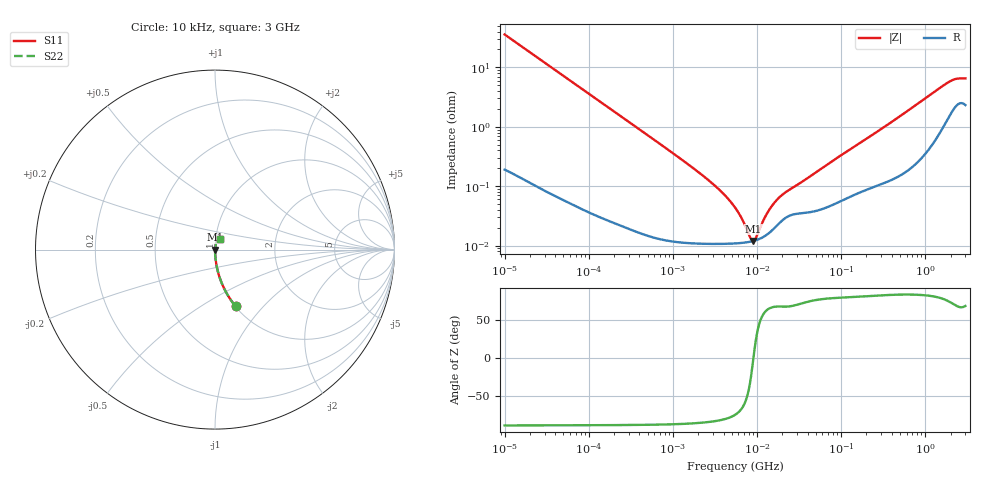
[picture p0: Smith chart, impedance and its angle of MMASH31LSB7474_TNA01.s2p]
! MMASH31LSB7474_TNA01  S-PARAMETER MODEL  ( Standard Model )
! Model Generated by TAIYO YUDEN Corporation (http://www.ty-top.com)
! Version 1.0
! TAIYO YUDEN Control No. 220601
! Copyright(c) 2013 TAIYO YUDEN CO.,LTD. All Rights Reserved.
! Product Description (link to TY-COMPAS)
! https://ds.yuden.co.jp/TYCOMPAS/or/detail?pn=MMASH31LSB7474KTNA01&u=M
! Products Name : Multilayer Ceramic Capacitors
! Characteristics :
!  Capacitance : 0.47 [uF] , Rated Voltage : 100 [V] , TCC : X7R
!  Case Size : 3.2 x 1.6 / 0.126 x 0.063 [mm/inch] , Thickness : 1.6 / 0.063 [mm/inch]
!  (Conditions: Temperature = 25 [degC] , DC Bias Voltage = 0 [V])
! External Node Assignments :
!  1  o---| |---o  2
! GND o---------o GND
! Frequency Range : 10kHz  -  3GHz  [ 401 STEP ]
# MHZ S RI R 50
! Freq[MHz].  S11 Real  S11 Imag  S21 Real  S21 Imag  S12 Real  S12 Imag  S22 Real  S22 Imag
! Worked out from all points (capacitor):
!   401 points, 10 kHz to 3 GHz, reference 50 ohm
!   read as one part in series: C = 445 nF near 10.65 kHz
!   lowest |Z| = 12 mohm at 9.071 MHz (marker M1)
!   series resonance near 9.072 MHz, so ESL is about 690 pH
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0.01  0.1143 -0.3155  0.8857 0.3155  0.8857 0.3155  0.1143 -0.3155
0.015549  0.0514 -0.2178  0.9486 0.2178  0.9486 0.2178  0.0514 -0.2178
0.026575  0.0187 -0.1322  0.9813 0.1322  0.9813 0.1322  0.0187 -0.1322
0.082683  0.0023 -0.0434  0.9977 0.0434  0.9977 0.0434  0.0023 -0.0434
0.683653  0.000158 -0.00529  0.9998 0.00529  0.9998 0.00529  0.000158 -0.00529
2.824956  0.000109 -0.00117  0.9999 0.00117  0.9999 0.00117  0.000109 -0.00117
4.124064  0.000108 -0.000705  0.9999 0.000705  0.9999 0.000705  0.000108 -0.000705
5.477226  0.000109 -0.000427  0.9999 0.000427  0.9999 0.000427  0.000109 -0.000427
6.617858  0.000112 -0.000261  0.9999 0.000261  0.9999 0.000261  0.000112 -0.000261
8.252149  0.000117 -7.76e-05  0.9999 7.76e-05  0.9999 7.76e-05  0.000117 -7.76e-05
8.789267  0.000119 -2.6e-05  0.9999 2.6e-05  0.9999 2.6e-05  0.000119 -2.6e-05
9.070798  0.00012 -1.39e-07  0.9999 1.39e-07  0.9999 1.39e-07  0.00012 -1.39e-07
9.97066  0.000125 7.77e-05  0.9999 -7.77e-05  0.9999 -7.77e-05  0.000125 7.77e-05
11.67315  0.000138 0.00021  0.9999 -0.00021  0.9999 -0.00021  0.000138 0.00021
13.24217  0.000155 0.000319  0.9998 -0.000319  0.9998 -0.000319  0.000155 0.000319
17.04125  0.000215 0.000539  0.9998 -0.000539  0.9998 -0.000539  0.000215 0.000539
21.93027  0.000295 0.000738  0.9997 -0.000738  0.9997 -0.000738  0.000295 0.000738
45.28751  0.000374 0.00151  0.9996 -0.00151  0.9996 -0.00151  0.000374 0.00151
374.4521  0.00135 0.0113  0.9986 -0.0113  0.9986 -0.0113  0.00135 0.0113
1811.492  0.0153 0.0513  0.9847 -0.0513  0.9847 -0.0513  0.0153 0.0513
2258.843  0.0241 0.057  0.9759 -0.057  0.9759 -0.057  0.0241 0.057
3000  0.0261 0.0581  0.9739 -0.0581  0.9739 -0.0581  0.0261 0.0581
